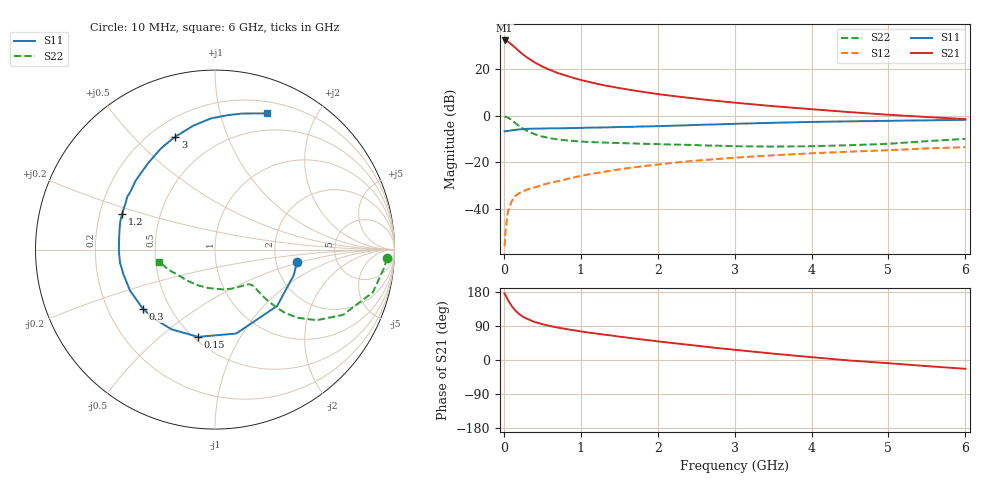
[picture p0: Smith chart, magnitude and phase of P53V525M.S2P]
! SIEMENS Small Signal Semiconductors
! BFP183
! Si NPN RF Bipolar Junction Transistor in SOT143
! VCE = 3.5 V  IC = 25 mA
! Common Emitter S-Parameters:  March  1996
# GHz  S  MA  R  50
!  f  S11  S21  S12  S22
! GHz  MAG  ANG  MAG  ANG  MAG  ANG  MAG  ANG
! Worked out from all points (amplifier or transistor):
!   36 points, 10 MHz to 6 GHz, reference 50 ohm
!   highest |S21| = 32.2 dB at 10 MHz (marker M1)
!   |S21| within 3 dB of that: start of sweep to 144.5 MHz
!   unconditionally stable (mu >= 1): 699.5 MHz to 5.658 GHz
!   at 250 MHz: K = 0.54, MSG = 29.3 dB, |S12| = -32.5 dB
!   at 1.4 GHz: K = 1.15, MAG = 15.6 dB, |S12| = -23.5 dB
!   at 6 GHz: K = 0.96, MSG = 6.0 dB, |S12| = -13.5 dB
!   S11 on the Smith chart (normalised r, x): 10 MHz: 2.62, -0.47; 150 MHz: 0.53, -0.68; 300 MHz: 0.35, -0.32; 1.2 GHz: 0.30, +0.17; 3 GHz: 0.29, +0.67; 6 GHz: 0.31, +1.41
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0.01  0.462 -8.7  40.6 175.7  0.0016 85.3  0.96 -2.9
0.02  0.4614 -17.9  40.49 171.8  0.0031 88.1  0.9479 -6.1
0.05  0.4674 -42.2  38.77 159.6  0.0084 78.3  0.9115 -15.1
0.1  0.4824 -75.8  33.32 143.0  0.0145 63.0  0.8009 -27.0
0.15  0.495 -100.9  28.22 130.3  0.0191 56.4  0.6894 -34.8
0.2  0.5056 -118.3  23.85 121.0  0.0219 53.4  0.5966 -39.5
0.25  0.5124 -130.6  20.3 114.0  0.0238 51.5  0.5274 -42.1
0.3  0.5199 -140.6  17.66 108.9  0.026 50.1  0.472 -43.3
0.4  0.5257 -154.4  13.8 100.4  0.0289 51.0  0.3997 -44.2
0.5  0.528 -164.4  11.23 94.6  0.0328 51.1  0.3562 -44.1
0.6  0.5341 -172.0  9.531 89.7  0.0364 52.9  0.3285 -43.8
0.7  0.5355 -178.6  8.164 85.7  0.0393 54.0  0.309 -43.5
0.8  0.5359 176.6  7.235 82.0  0.0429 54.9  0.296 -43.6
1.1  0.5512 163.0  5.295 72.4  0.0551 55.4  0.2722 -45.2
1.2  0.5539 159.1  4.848 69.9  0.0585 55.3  0.2684 -46.1
1.7  0.5767 142.5  3.417 56.6  0.0784 53.7  0.2531 -53.3
2.2  0.6071 128.4  2.626 44.6  0.0976 50.1  0.2397 -63.2
3  0.6667 109.4  1.893 27.0  0.1254 42.8  0.2211 -83.9
3.5  0.701 99.9  1.592 16.8  0.141 38.4  0.2172 -99.1
4.5  0.7529 84.4  1.185 -1.4  0.1689 29.2  0.2322 -131.8
5.5  0.791 73.6  0.932 -16.1  0.198 21.2  0.2835 -156.9
6  0.8129 69.0  0.841 -23.2  0.2106 16.6  0.3173 -167.7
